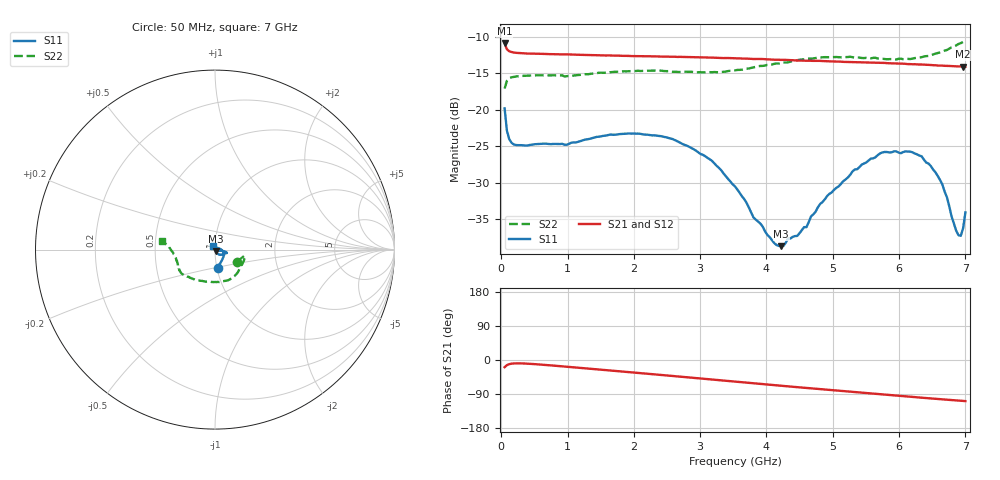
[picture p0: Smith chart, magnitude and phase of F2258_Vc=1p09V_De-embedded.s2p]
! Integrated Device Technology
! Corporate Headquarters
! 6024 Silver Creek Valley Road
! San Jose, CA 95138  USA
! Phone:  1-408-284-8200
! Toll Free:  1-800-223-1366
! Webpage:  http://www.idt.com/
! Timing and RF Division
! 515 Groton Road, Suite 102
! Westford, MA 01886-6024
! Device:  F2258
! Description: Voltage Variable RF Attenuator
! Frequency:  50.0 -  6000.00 MHz
! Package:  3x3 mm Thin QFN Plastic Package: 16 pin
! Ports:  2 RF, 2 DC
!  Pin  1  = NC
!  Pin  2  = NC
!  Pin  3  = RF2  = Port 2
!  Pin  4  = GND
!  Pin  5  = Vdd
!  Pin  6  = NC
!  Pin  7  = VCTRL
!  Pin  8  = NC
!  Pin  9  = GND
!  Pin 10  = RF1  = Port 1
!  Pin 11  = NC
!  Pin 12  = NC
!  Pin 13  = NC
!  Pin 14  = NC
!  Pin 15  = NC
!  Pin 16  = NC
! Vcntrl:  1.090 Volts
! Vdd:  +3.300 Volts
! Current:  1.161 mA
! Data:  The device was measured on a the F2258 evaluation board which has
!  individual transmission lines to the RF pins.  Data was collected
!  using a calibrated network analyzer.  The evaluation board was
!  de-embedded using a TRL calibration technique.
!  The reference plane is the edge of the package pin.
! Misc:  SN 10
!  Action Tracker AT0285
! Date Measured:  2014-12-10
! Date:  2016-01-13  MJV
! Note:
!  Integrated Device Technology supplies this data as a sample of measured
!  data at the package pin for this product.  Your particular data for this
!  product may vary.
!  Data was taken at 25 degrees C.
!  Integrated Device Technology reserves the right to change this data at anytime.
!Freq_(GHz)  S11M_(dB)  S11P_(deg)  S21M_(dB)  S21P_(deg)  S12M_(dB)  S12P_(deg)  S22M_(dB)  S22P_(deg)
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# GHz S dB R 50
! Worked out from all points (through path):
!   201 points, 50 MHz to 7 GHz, reference 50 ohm
!   highest |S21| = -10.89 dB at 50 MHz (marker M1); lowest = -14.1 dB at 6.965 GHz (marker M2)
!   group delay of S21, straight-line fit = 41.9 ps
!   lowest |S11| = -38.7 dB at 4.22 GHz (marker M3), VSWR 1.02, Z = 50.7 - j0.921 ohm
!   |S11| at or under -10 dB: start of sweep to end of sweep
!   |S22| runs from -17.1 to -10.5 dB; largest |S21 - S12| = 0.0017
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0.05  -19.80 -81.9  -10.89 -19.0  -10.90 -19.0  -17.09 -28.4
0.08475  -22.85 -58.4  -11.71 -13.5  -11.72 -13.5  -16.02 -15.8
0.1195  -24.01 -43.4  -11.97 -11.0  -11.97 -11.0  -15.69 -12.7
0.189  -24.75 -28.8  -12.15 -9.1  -12.17 -9.1  -15.48 -11.4
1.2315  -24.17 -17.7  -12.47 -21.4  -12.48 -21.4  -15.16 -38.4
1.9265  -23.24 -15.1  -12.62 -32.0  -12.66 -32.0  -14.71 -55.9
2.37825  -23.58 -13.0  -12.70 -38.9  -12.74 -38.9  -14.64 -67.7
3.07325  -26.33 -10.7  -12.82 -49.9  -12.86 -49.8  -14.86 -90.4
3.525  -30.50 -12.6  -12.95 -57.0  -12.97 -57.0  -14.60 -108.1
3.803  -34.73 -22.1  -13.04 -61.4  -13.02 -61.5  -14.18 -119.0
4.11575  -38.25 -41.9  -13.13 -66.3  -13.13 -66.3  -13.71 -128.7
4.22  -38.68 -51.2  -13.16 -67.9  -13.14 -67.9  -13.59 -131.6
4.60225  -36.07 -69.3  -13.28 -73.7  -13.28 -73.7  -12.99 -140.0
4.7065  -34.32 -65.6  -13.30 -75.3  -13.30 -75.3  -12.97 -141.8
5.332  -28.17 -45.5  -13.47 -84.6  -13.46 -84.6  -12.87 -151.1
5.85325  -25.84 -29.8  -13.62 -92.3  -13.63 -92.3  -13.06 -160.9
6.33975  -26.36 -15.1  -13.80 -99.5  -13.82 -99.5  -12.79 -173.1
6.6525  -30.23 5.1  -13.94 -103.8  -13.99 -103.7  -12.02 178.6
6.89575  -37.18 70.5  -14.06 -107.1  -14.09 -107.1  -10.99 172.7
6.9305  -37.25 86.0  -14.06 -107.5  -14.11 -107.5  -10.86 172.3
6.96525  -36.24 103.9  -14.10 -108.1  -14.12 -108.0  -10.70 171.3
7  -34.04 116.2  -14.10 -108.5  -14.13 -108.5  -10.50 170.4
